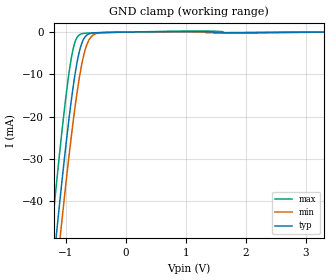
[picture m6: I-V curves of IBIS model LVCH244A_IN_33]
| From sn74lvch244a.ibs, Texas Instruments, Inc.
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[Model]   LVCH244A_IN_33
Model_type  Input
Vinl=0.8
Vinh=2.0
| variable   typ   min   max
C_comp   3.42pF   3.03pF   3.96pF
[Temperature Range]   40   100   -40
| Ambient temperature   25   85   -40
[Voltage range]   3.3   3   3.6
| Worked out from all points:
|   GND clamp passes 1 mA (typ) near -0.67 V on its own axis
[GND Clamp]
| LVCH244A_IN_33
|   Voltage   I(typ)   I(min)   I(max)
-5.5V     -733.1mA   -739.5mA   -725.5mA
-1.25V    -61.03mA   -70.25mA   -49.21mA
-1.22V    -56.74mA   -65.97mA   -44.88mA
-1.145V   -46.18mA   -55.43mA   -34.27mA
-1.095V   -39.32mA   -48.55mA   -27.46mA
-1.075V   -36.64mA   -45.85mA   -24.81mA
-950mV    -20.83mA   -29.66mA   -9.971mA
-855mV    -10.73mA   -18.65mA   -2.714mA
-775mV    -4.615mA   -10.83mA   -646.3uA
-705mV    -1.698mA   -5.678mA   -296.5uA
-555mV    -211.3uA   -801.5uA   -183.2uA
3.3V      1.12nA     84.83nA    -89.12nA
